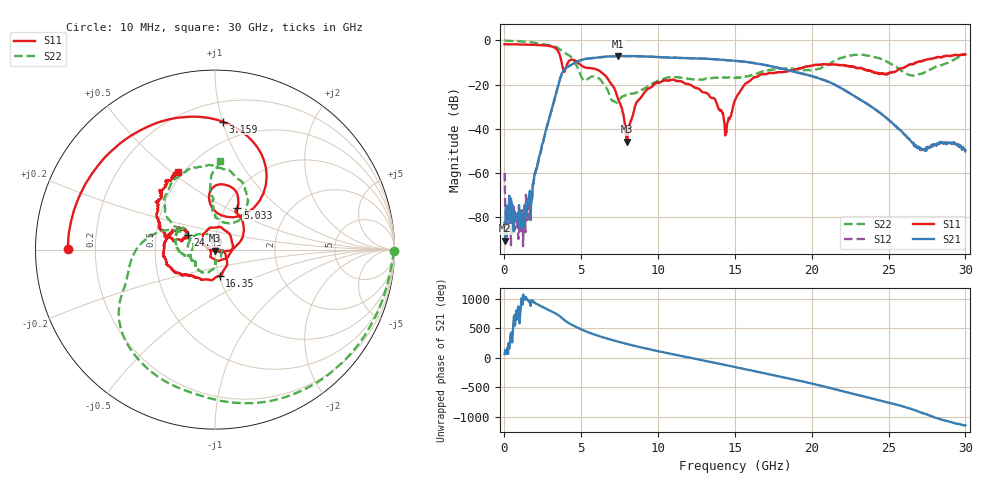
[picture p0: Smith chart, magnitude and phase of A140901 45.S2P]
!  2-Port S-parameters saved by WinCal
! VAR MeasName=S-Parameters (CALIBRATED_DATA) read from VNA (N5244A)
! VAR MeasDate=11/3/2014 9:34:07 AM
! VAR NAME=A140901 45
! VAR FILENAME=A140901 45.S2P
! VAR DATE=11/3/2014 9:34:07 AM
! VAR PHYS_PORTS=1,2
# Hz S RI R 50
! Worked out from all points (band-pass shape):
!   801 points, 10 MHz to 30 GHz, reference 50 ohm
!   highest |S21| = -7.08 dB at 7.395 GHz (marker M1); lowest = -90.8 dB at 47.49 MHz (marker M2)
!   |S21| within 3 dB of the highest: 4.609 GHz to 16.08 GHz (11.48 GHz wide, 111 % of centre)
!   lowest |S11| = -45.9 dB at 7.957 GHz (marker M3), VSWR 1.01, Z = 50.1 - j0.506 ohm
!   |S11| at or under -10 dB: 3.724 GHz to 4.134 GHz (409.8 MHz wide, 10.4 % of centre); 4.771 GHz to 26.77 GHz (22 GHz wide, 139 % of centre); 26.78604 GHz to 26.82312 GHz (37.07 MHz wide, 0.138 % of centre)
!   |S22| runs from -28.2 to 0.0 dB; largest |S21 - S12| = 0.0026
!   S11 on the Smith chart (normalised r, x): 10 MHz: 0.10, +0.00; 3.159 GHz: 0.34, +1.00; 5.033 GHz: 1.13, +0.57; 16.35 GHz: 1.01, -0.30; 24.49 GHz: 0.73, +0.12; 30 GHz: 0.47, +0.53
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1e7  -0.8188 0.00286  3.17e-05 6.62e-05  0.000622 0.000775  0.9986 -0.00823
4.74875e7  -0.8188 0.0151  -1.92e-05 2.13e-05  0.000172 7.74e-06  0.9925 -0.0375
2.34925e8  -0.8155 0.0765  5.38e-05 0.000134  1.03e-05 8.38e-05  0.9699 -0.1546
1.35955e9  -0.6854 0.4232  1.14e-05 -0.000123  -3.89e-05 -2.23e-05  0.5995 -0.7197
3.15895e9  0.0421 0.7132  0.0186 0.0289  0.0186 0.0287  -0.4149 -0.6248
3.871212e9  0.0641 0.1828  0.0661 -0.2055  0.0667 -0.2047  -0.4992 -0.1916
5.033325e9  0.1251 0.2336  -0.1767 0.3178  -0.1769 0.3177  -0.1316 0.0542
6.195438e9  0.1602 0.1241  0.4139 0.046  0.4132 0.0464  -0.1052 0.0824
7.395038e9  0.0445 -0.0133  0.0316 -0.4415  0.0324 -0.4413  0.0359 -0.0178
7.95735e9  0.000531 -0.00505  -0.2474 -0.3655  -0.2469 -0.366  0.0148 -0.056
8.669612e9  -0.0412 0.00872  -0.4323 -0.0789  -0.4321 -0.079  0.00362 -0.0677
1.001916e10  -0.0606 0.0916  -0.1519 0.3919  -0.1509 0.3906  -0.0288 -0.1209
1.215595e10  0.0965 0.00234  0.394 -0.0262  0.3934 -0.0248  -0.1099 -0.0743
1.365545e10  -0.0259 -0.0404  0.0379 -0.3727  0.0387 -0.373  -0.1294 -0.0612
1.44052e10  -0.00375 0.00791  -0.2022 -0.2958  -0.2016 -0.2962  -0.1368 -0.04
1.5005e10  0.0437 -0.00515  -0.3172 -0.1359  -0.3167 -0.1365  -0.1376 -0.0321
1.635455e10  0.0266 -0.1449  -0.1849 0.2378  -0.1872 0.2373  -0.1692 -0.0313
2.002832e10  -0.2509 -0.0969  0.0269 -0.1513  0.0274 -0.152  -0.1748 0.1122
2.448934e10  -0.1512 0.0826  0.0219 -0.00366  0.0219 -0.00344  0.1678 0.3427
2.501416e10  -0.1638 0.0642  0.0114 -0.0109  0.0113 -0.0108  0.1823 0.258
2.711346e10  -0.3036 0.1317  -0.00294 0.0018  -0.00277 0.00168  0.00768 0.1763
3e10  -0.2081 0.4324  0.00125 -0.00303  0.000795 -0.00276  0.0276 0.493
